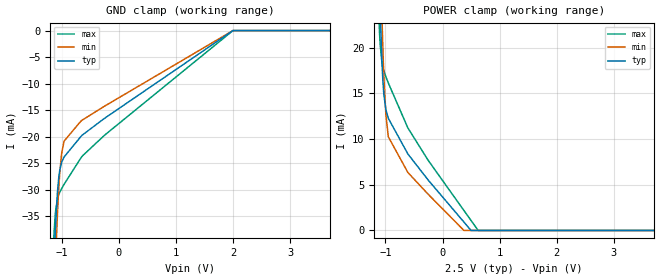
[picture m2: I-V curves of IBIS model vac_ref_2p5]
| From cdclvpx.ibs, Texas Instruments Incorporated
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|   Vac_ref_2p5 Model   |
[Model]   vac_ref_2p5
Model_type   Terminator
|   typ   min   max
|   (nom PVT)   (fast PVT)   (slow PVT)
C_comp   1.498e-13   1.487e-13   1.517e-13
| Where nom  PVT is Nominal Process, 2.5V, 40C
|   Fast PVT is Strong Process,  2.625V, -40C
|   Slow PVT is Weak Process,   2.375V,100C
[Voltage Range]   2.5   2.375   2.625
|Junction Temperature
[Power Clamp Reference]   2.5   2.375   2.625
[GND Clamp Reference]   0   0   0
[GND Clamp]
|   Voltage   I(typ)   I(min)   I(max)
-2.5V     -688.6mA   -693.5mA   -686.1mA
-1.134V   -44.07mA   -51.79mA   -38.21mA
-1.111V   -37.65mA   -44.26mA   -34.43mA
-1.105V   -36.32mA   -42.59mA   -33.81mA
-1.075V   -30.58mA   -34.66mA   -31.72mA
-1.052V   -27.79mA   -29.9mA    -30.92mA
-1.035V   -26.39mA   -27.01mA   -30.48mA
-1.002V   -24.85mA   -23.27mA   -29.8mA
-958.6mV  -23.82mA   -20.83mA   -28.96mA
-665mV    -19.97mA   -17.07mA   -24.01mA
1.998V    -15.61uA   -11.08uA   -15.33uA
5V        0A         0A         0A
[POWER Clamp]
|   Voltage   I(typ)   I(min)   I(max)
-2.5V     683mA      688.9mA    679.5mA
-1.123V   32.1mA     40.97mA    24.77mA
-1.103V   26.88mA    34.88mA    21.64mA
-1.093V   24.23mA    31.59mA    20.39mA
-1.062V   18.45mA    23.46mA    18.41mA
-1.032V   15.26mA    17.66mA    17.58mA
-992.5mV  13.22mA    12.7mA     16.83mA
-949.1mV  12.27mA    10.25mA    16.14mA
-607.4mV  8.381mA    6.351mA    11.23mA
373.8mV   927.5uA    7.912uA    2.201mA
625mV     0A         0A         8.345uA
5V        0A         0A         0A
